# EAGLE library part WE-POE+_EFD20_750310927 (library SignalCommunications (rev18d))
WE-PoE+ Power over Ethernet Plus Transformer Characteristics Designed to meet 25 W PoE+ requirements of IEEE802.3at Frequency range: 250–400 kHz Input voltage range: 36–72 V 1.5 kV Hipot test between primary and secondary Operating temperature: –40 °C to +125 °C Applications PoE+ powered devices IP phones WLAN-Access points Security cameras Details see: http://katalog.we-online.de/en/pbs/WE-POE-PLUS?m Updated by Dan Xu 2014-07-08 2014 (C) Wurth Elektronik
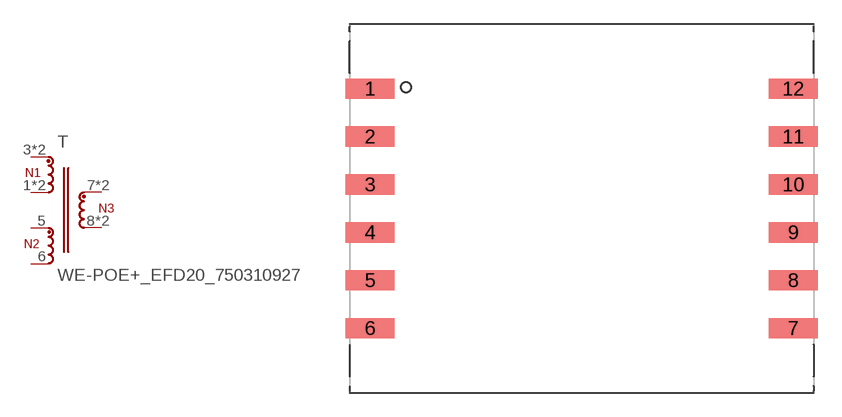
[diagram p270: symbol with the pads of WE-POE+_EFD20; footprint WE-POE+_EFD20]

Designator prefix T

## WE-POE+_EFD20_750310927  [WE-POE+_EFD20]
1  2  pas
2  2  pas
3  1  pas
4  1  pas
5  3  pas
6  4  pas
7  6  pas
8  5  pas
9  6  pas
10  5  pas

## Footprint WE-POE+_EFD20 (pad centres in mm)
Transformer, EFD20 SMD 12 Pin
smd 3.05 x 1.27: 1 -13.26,7.5; 2 -13.26,4.5; 3 -13.26,1.5; 4 -13.26,-1.5; 5 -13.26,-4.5; 6 -13.26,-7.5; 7 13.26,-7.5; 8 13.26,-4.5; 9 13.26,-1.5; 10 13.26,1.5; 11 13.26,4.5; 12 13.26,7.5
